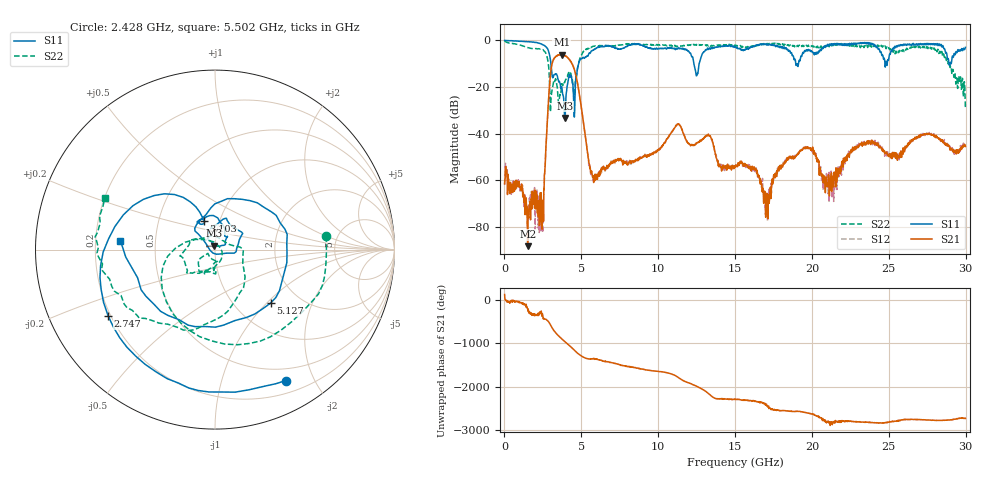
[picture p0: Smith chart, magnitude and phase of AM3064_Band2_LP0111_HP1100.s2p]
# Hz S DB R 50.0
!freq dBS11 angS11 dBS21 angS21 dBS12 angS12 dBS22 angS22
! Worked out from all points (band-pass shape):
!   1600 points, 10 MHz to 29.98 GHz, reference 50 ohm
!   highest |S21| = -6.10 dB at 3.721 GHz (marker M1); lowest = -88.4 dB at 1.51 GHz (marker M2)
!   |S21| within 3 dB of the highest: 3.137 GHz to 4.317 GHz (1.18 GHz wide, 31.6 % of centre)
!   lowest |S11| = -33.4 dB at 3.946 GHz (marker M3), VSWR 1.04, Z = 49.6 + j2.11 ohm
!   |S11| at or under -10 dB: 3.02 GHz to 4.825 GHz (1.805 GHz wide, 46 % of centre); 12.32 GHz to 12.66 GHz (342.7 MHz wide, 2.74 % of centre); 18.95 GHz to 19.12 GHz (176.8 MHz wide, 0.929 % of centre)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
!   |S22| runs from -30.7 to -0.2 dB; largest |S21 - S12| = 0.013
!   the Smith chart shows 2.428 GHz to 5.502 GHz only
!   S11 on the Smith chart (normalised r, x): 2.428 GHz: 0.35, -1.62; 2.747 GHz: 0.19, -0.27; 3.103 GHz: 0.84, +0.28; 5.127 GHz: 1.44, -1.05; 5.502 GHz: 0.31, +0.04
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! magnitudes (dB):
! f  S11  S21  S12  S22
! 10 MHz  -0.1  -61.6  -62.0  -0.2
! 1.51 GHz  -0.6  -88.4  -75.0  -3.1
! 2.428 GHz  -1.6  -73.2  -70.1  -4.1
! 2.747 GHz  -3.1  -39.7  -39.9  -6.5
! 3.103 GHz  -15.3  -9.8  -9.9  -21.2
! 3.721 GHz  -19.9  -6.1  -6.1  -18.6
! 3.946 GHz  -33.4  -6.5  -6.5  -17.4
! 5.015 GHz  -7.9  -29.5  -29.5  -6.4
! 5.127 GHz  -7.3  -34.8  -34.9  -4.9
! 5.502 GHz  -5.5  -52.8  -53.1  -3.4
! 10 GHz  -3.6  -47.3  -46.9  -2.0
! 11.31 GHz  -3.2  -36.1  -36.0  -2.6
! 12.49 GHz  -15.2  -44.1  -44.3  -2.0
! 15 GHz  -2.7  -54.3  -53.8  -2.1
! 16.3 GHz  -2.2  -55.0  -56.2  -2.3
! 17.05 GHz  -2.0  -73.4  -71.6  -1.5
! 19.99 GHz  -4.6  -46.8  -46.8  -2.3
! 21.27 GHz  -1.4  -56.9  -61.4  -2.2
! 23.05 GHz  -1.1  -45.4  -44.1  -2.7
! 25 GHz  -8.1  -49.7  -49.1  -3.2
! 28.31 GHz  -2.2  -42.6  -42.9  -4.7
! 29.98 GHz  -3.0  -45.6  -45.5  -29.2
